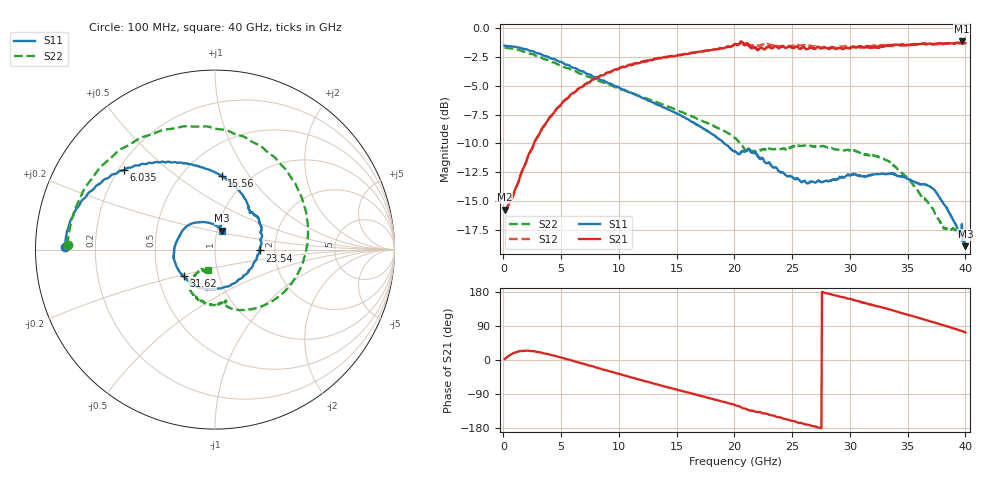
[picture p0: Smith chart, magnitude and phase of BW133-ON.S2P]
!  2-Port S-parameters saved by WinCal
! VAR MeasName=S-Parameters (CALIBRATED_DATA) read from VNA (N5244A)
! VAR MeasDate=2013-8-7 14:07:32
! VAR NAME=136504 2
! VAR FILENAME=136504 2.S2P
! VAR DATE=2013-8-7 14:07:32
! VAR PHYS_PORTS=1,2
# Hz S MA R 50
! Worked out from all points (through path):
!   801 points, 100 MHz to 40 GHz, reference 50 ohm
!   highest |S21| = -1.14 dB at 39.7 GHz (marker M1); lowest = -15.7 dB at 100 MHz (marker M2)
!   lowest |S11| = -18.9 dB at 40 GHz (marker M3), VSWR 1.26, Z = 52.9 + j11.4 ohm
!   |S11| at or under -10 dB: 19.14 GHz to end of sweep
!   |S22| runs from -18.5 to -1.7 dB; largest |S21 - S12| = 0.05
!   S11 on the Smith chart (normalised r, x): 100 MHz: 0.09, +0.01; 6.035 GHz: 0.22, +0.36; 15.56 GHz: 0.76, +0.75; 23.54 GHz: 1.66, -0.02; 31.62 GHz: 0.68, -0.21; 40 GHz: 1.06, +0.23
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1e8  0.8374 179.2  0.1636 2.6  0.163 2.5  0.8218 178.1
1.346875e9  0.8228 169.3  0.2192 22.9  0.218 22.9  0.8029 155.5
3.142375e9  0.7743 156.3  0.35 20.4  0.3478 20.7  0.7502 124.7
4.489e9  0.7294 147.6  0.4387 10.8  0.4371 11.3  0.705 102.8
6.035125e9  0.6725 138.8  0.524 -2.6  0.52 -1.8  0.6519 78.9
6.78325e9  0.6504 134.7  0.5547 -9.0  0.5538 -8.1  0.6316 67.7
8.2795e9  0.6012 126.5  0.617 -21.7  0.6166 -21.0  0.589 45.7
9.925375e9  0.5555 118.2  0.6613 -36.0  0.6664 -35.1  0.55 23.2
1.341662e10  0.4635 99.1  0.7387 -65.4  0.7411 -64.6  0.4745 -19.5
1.556125e10  0.4125 84.8  0.7665 -82.3  0.7696 -81.8  0.4301 -41.5
1.760612e10  0.3604 69.4  0.7982 -99.0  0.7974 -98.1  0.3894 -58.8
2.005e10  0.2932 49.0  0.8537 -119.0  0.8441 -117.5  0.334 -75.9
2.114725e10  0.2999 38.6  0.8573 -131.3  0.8514 -128.7  0.2947 -78.1
2.354125e10  0.2492 -1.1  0.8345 -148.3  0.8413 -148.4  0.2989 -82.4
2.673325e10  0.2166 -59.0  0.8166 -174.1  0.8276 -174.1  0.3075 -94.2
2.9227e10  0.2261 -102.8  0.8172 166.6  0.8254 167.4  0.2943 -103.7
3.1621e10  0.2295 -139.8  0.8348 147.1  0.8305 148.6  0.281 -113.0
3.336662e10  0.2344 -164.0  0.8381 133.8  0.8379 133.6  0.265 -121.7
3.715712e10  0.2022 138.6  0.8518 100.6  0.8471 100.8  0.165 -127.5
3.810475e10  0.1734 118.8  0.8559 91.6  0.8507 92.8  0.1358 -121.5
3.970075e10  0.1418 75.9  0.8773 76.6  0.8824 77.5  0.1308 -124.5
4e10  0.1137 69.2  0.8602 72.9  0.8571 73.4  0.1185 -109.0
